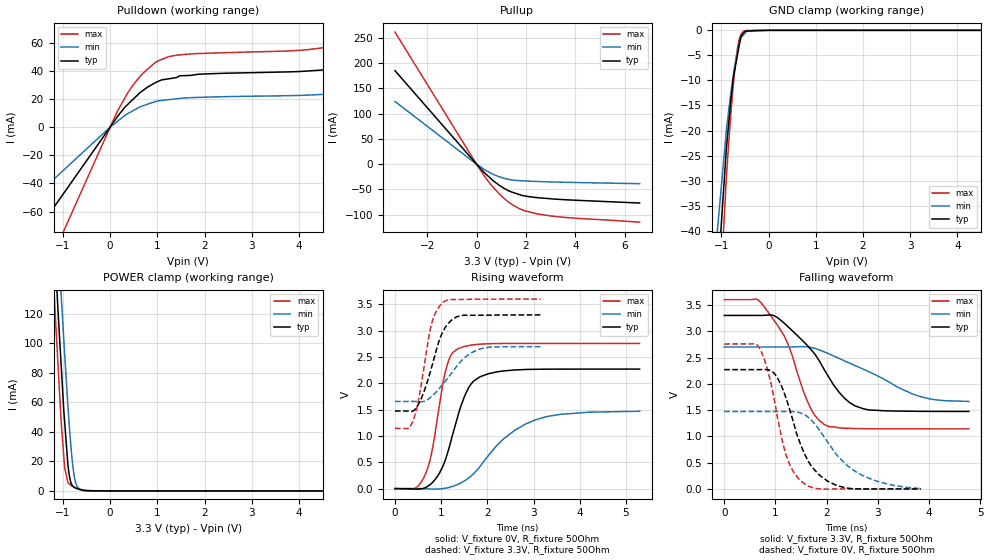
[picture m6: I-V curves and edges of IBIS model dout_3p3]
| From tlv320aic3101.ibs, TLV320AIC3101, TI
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|   dout_3p3 Model
[Model]   dout_3p3
Model_type   3-state
Polarity   Non-Inverting
Vmeas = 1.65
Vref = 1.65
Cref = 10pF
Rref = 50
|   typ   min   max
|   (nom PVT)   (fast PVT)   (slow PVT)
 C_comp   1.458e-12   1.424e-12   1.523e-12
| Where nom  PVT is Nominal Process, 3.3V, 27C
|   Fast PVT is Strong Process,  3.6V, -40C
|   Slow PVT is Weak Process,   2.7V, 105C
[Voltage Range]   3.3   2.7   3.6
|Ambient Temperature   25   85   -40
|Junction Temperature
[Temperature Range]   27   105   -40
[Pullup Reference]   3.3   2.7   3.6
[Pulldown Reference]   0   0   0
[Power Clamp Reference]   3.3   2.7   3.6
[GND Clamp Reference]   0   0   0
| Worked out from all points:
|   slope of the pulldown table from 0 to 0.495 V, typ, clamps not added: 24.6 ohm
|   slope of the pullup table from 0 to 0.495 V, typ, clamps not added: 19.9 ohm
|   GND clamp passes 1 mA (typ) near -0.57 V on its own axis
|   POWER clamp passes 1 mA (typ) near -0.64 V on its own axis
|   falling waveform, V_fixture 3.3V, R_fixture 50Ohm: 20-80 % time 834ps typ, 1.31ns min, 596ps max; typ from 3.3 V to 1.48 V
|   rising waveform, V_fixture 0V, R_fixture 50Ohm: 20-80 % time 487ps typ, 1.01ns min, 326ps max; typ from 0 V to 2.27 V
|   rising waveform, V_fixture 3.3V, R_fixture 50Ohm: 20-80 % time 386ps typ, 590ps min, 289ps max; typ from 1.47 V to 3.3 V
|   falling waveform, V_fixture 0V, R_fixture 50Ohm: 20-80 % time 515ps typ, 808ps min, 379ps max; typ from 2.27 V to 0 V
[Pulldown]
|   Voltage   I(typ)   I(min)   I(max)
-3.3V     -157.7mA   -102.3mA   -247.6mA
-132.3mV  -6.322mA   -4.101mA   -9.925mA
154.8mV   7.524mA    4.153mA    11.4mA
385.2mV   16.6mA     9.851mA    25.06mA
684mV     25.82mA    15.04mA    38.01mA
1.008V    32.39mA    18.58mA    47.01mA
1.595V    36.65mA    20.77mA    51.78mA
4.162V    39.88mA    22.75mA    54.99mA
5.145V    44.71mA    26.5mA     63mA
5.666V    52.1mA     29.08mA    74.5mA
6.376V    71.54mA    32.6mA     104.4mA
6.6V      80.7mA     33.72mA    118.2mA
[GND Clamp]
|   Voltage   I(typ)   I(min)   I(max)
-3.3V     -1.433A    -1.242A    -1.601A
-1.501V   -109.4mA   -83.8mA    -137.1mA
-897.6mV  -23.87mA   -20.19mA   -29.72mA
-842.4mV  -18.16mA   -15.67mA   -21.99mA
-772.2mV  -11.49mA   -10.54mA   -13.43mA
-702mV    -7.044mA   -6.238mA   -6.494mA
-622.8mV  -2.919mA   -2.734mA   -1.801mA
-590.7mV  -1.247mA   -1.753mA   -932.8uA
-532.8mV  -547.5uA   -921.6uA   -189.6uA
-464.4mV  -157.9uA   -173uA     -21.1uA
-286.2mV  -97.29uA   -2.289uA   -5.49uA
6.6V      0A         0A         0A
[Pullup]
|   Voltage   I(typ)   I(min)   I(max)
-3.3V     185.2mA    124.3mA    261.7mA
136.8mV   -7.535mA   -4.589mA   -10.54mA
633.6mV   -31.13mA   -19.16mA   -43.6mA
939.6mV   -42.5mA    -25.4mA    -59.94mA
1.246V    -51.46mA   -29.66mA   -73.23mA
1.447V    -55.61mA   -31.4mA    -80.33mA
1.861V    -62.28mA   -33.04mA   -90.87mA
2.437V    -66.24mA   -34.26mA   -98.47mA
3.701V    -70.81mA   -36.05mA   -106mA
6.6V      -77.05mA   -38.71mA   -115mA
[POWER Clamp]
|   Voltage   I(typ)   I(min)   I(max)
-3.3V     1.575A     1.59A      1.584A
-1.287V   233mA      282mA      198.3mA
-1.166V   159.5mA    208.2mA    121.1mA
-1.118V   129.8mA    179.3mA    92.94mA
-1.037V   84.49mA    132.4mA    46.22mA
-964.8mV  46.89mA    93.07mA    15.88mA
-881.1mV  13.91mA    51.04mA    5.244mA
-801.9mV  3.543mA    19.94mA    3.226mA
-745.8mV  2.064mA    7.584mA    2.255mA
-669.6mV  1.298mA    1.804mA    1.176mA
-334.8mV  127.1uA    7.167uA    265nA
6.6V      0A         0A         0A
[Ramp]
R_load = 50
|   typ   min   max
dV/dt_r   1.36197/4.86473e-10   0.883866/1.00875e-09   1.65397/3.25684e-10
dV/dt_f   1.09591/8.34062e-10   0.626508/1.315e-09   1.47417/5.95402e-10
[Falling Waveform]
V_fixture = 3.3V
V_fixture_min = 2.7V
V_fixture_max = 3.6V
R_fixture = 50Ohm
|   Time   V(typ)   V(min)   V(max)
0s        3.3V       2.7V       3.6V
622ps     3.3V       2.7V       3.611V
736ps     3.3V       2.7V       3.523V
1.16ns    3.163V     2.7V       2.93V
1.626ns   2.726V     2.702V     1.663V
1.964ns   2.251V     2.603V     1.222V
2.344ns   1.73V      2.438V     1.154V
2.716ns   1.526V     2.278V     1.147V
3.832ns   1.477V     1.756V     1.144V
4.776ns   1.475V     1.665V     1.143V
[Rising Waveform]
V_fixture = 0V
V_fixture_min = 0V
V_fixture_max = 0V
R_fixture = 50Ohm
|   Time   V(typ)   V(min)   V(max)
0s        1.435nV    19.75nV    865pV
418ps     -7.496mV   161.4uV    -222.2uV
640ps     11.96mV    -3.273mV   237.8mV
796ps     103.7mV    -7.576mV   689.2mV
1.086ns   534.6mV    6.839mV    2.201V
1.36ns    1.373V     79.36mV    2.656V
1.646ns   1.986V     237.5mV    2.725V
2.024ns   2.182V     630.5mV    2.752V
3.034ns   2.266V     1.304V     2.756V
5.296ns   2.27V      1.469V     2.757V
[Rising Waveform]
V_fixture = 3.3V
V_fixture_min = 2.7V
V_fixture_max = 3.6V
R_fixture = 50Ohm
|   Time   V(typ)   V(min)   V(max)
0s        1.473V     1.656V     1.143V
278ps     1.473V     1.656V     1.14V
394ps     1.476V     1.656V     1.293V
518ps     1.617V     1.651V     1.722V
766ps     2.222V     1.73V      3.035V
868ps     2.544V     1.815V     3.321V
1.002ns   2.914V     1.945V     3.507V
1.33ns    3.26V      2.317V     3.591V
1.77ns    3.292V     2.63V      3.597V
3.154ns   3.299V     2.696V     3.6V
[Falling Waveform]
V_fixture = 0V
V_fixture_min = 0V
V_fixture_max = 0V
R_fixture = 50Ohm
|   Time   V(typ)   V(min)   V(max)
0s        2.27V      1.473V     2.757V
684ps     2.27V      1.473V     2.686V
878ps     2.263V     1.473V     2.15V
1.038ns   2.113V     1.473V     1.365V
1.198ns   1.754V     1.473V     675.5mV
1.354ns   1.263V     1.471V     323.2mV
1.57ns    663.9mV    1.41V      97.41mV
2.006ns   158.2mV    911.1mV    -3.05mV
2.556ns   1.577mV    336.2mV    728.7uV
3.84ns    428.8uV    8.222mV    91.34uV
